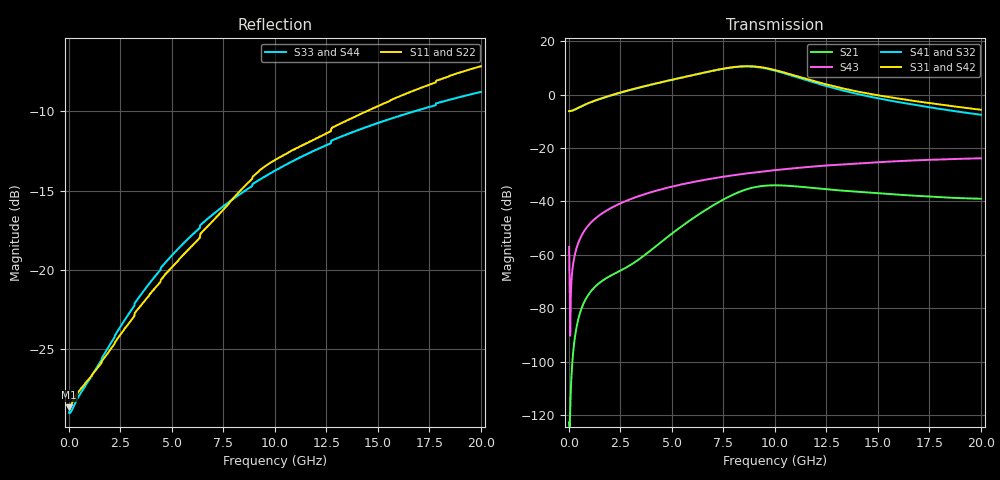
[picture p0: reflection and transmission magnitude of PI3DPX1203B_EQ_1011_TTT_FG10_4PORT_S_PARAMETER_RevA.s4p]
! NPort=4 DATA=2000 NOISE=0 GROUPDELAY=0 COMPLEX_DATAFORMAT=POLAR
! NumOfBlock=1 NumOfParam=0
! .MODEL Smodel S TSTONEFILE=PI3DPX1203B_EQ_1011_TTT_FG10_4PORT_S_PARAMETER_RevA.s4p TYPE=S
!  -- The above .MODEL line can be used for the S element in the netlist.
! The s parameter is extracted from the linear redriver, it is not bi-directional; only s(4,1)s(4,2) and s(3,1)s(3,2)
! should be the insertion loss
!Port definition:
!Port1 = input+
!Port2 = input-
!Port3 = output+
!Port4 = output-
# Hz S MA R  50
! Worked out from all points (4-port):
!   2000 points, 10 MHz to 20 GHz, reference 50 ohm
!   strongest paths, dB at 10 MHz, 5.01 GHz, 10.01 GHz, 15.01 GHz, 20 GHz:
!     S31: -6.2, 5.6, 9.2, -0.3, -5.7
!     S42: -6.2, 5.6, 9.2, -0.3, -5.7
!     S41: -6.2, 5.6, 9.0, -1.4, -7.6
!     S32: -6.2, 5.6, 9.0, -1.4, -7.6
!     S43: -57.1, -34.4, -28.3, -25.3, -23.8
!     S21: -122.7, -52.0, -34.0, -37.0, -39.0
!   lowest |S11| = -28.6 dB at 10 MHz (marker M1), VSWR 1.08, Z = 46.4 - j0.0306 ohm
!   |S11| at or under -10 dB: start of sweep to 14.45 GHz
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1e7  0.03701 -179.5  7.338e-07 10.7  0 0.0  0 0.0
     7.338e-07 10.7  0.03701 -179.5  0 0.0  0 0.0
     0.4917 -0.0  0.4917 180.0  0.03566 178.2  0.001403 -77.8
     0.4917 180.0  0.4917 -0.0  0.001403 -77.8  0.03566 178.2
3.08e9  0.07029 -126.9  0.0006803 139.5  1.482e-10 56.1  2.591e-09 107.3
        0.00068 139.5  0.07029 -126.9  2.591e-09 107.3  1.482e-10 56.1
        1.262 1.7  1.25 -177.1  0.07565 -126.7  0.01139 77.7
        1.25 -177.1  1.262 1.7  0.01139 77.7  0.07565 -126.7
5.82e9  0.1163 -111.0  0.004264 153.6  1.23e-08 -121.2  1.123e-07 69.2
        0.004263 153.6  0.1163 -111.0  1.123e-07 69.2  1.23e-08 -121.2
        2.235 -39.7  2.234 141.7  0.1263 -117.3  0.02225 66.0
        2.234 141.7  2.235 -39.7  0.02225 66.0  0.1263 -117.3
8.21e9  0.1749 -105.0  0.01475 111.0  3.09e-07 156.0  8.63e-07 20.0
        0.01474 111.0  0.1749 -105.0  8.622e-07 20.0  3.092e-07 156.0
        3.347 -98.7  3.316 82.5  0.1716 -115.9  0.03183 53.9
        3.317 82.5  3.346 -98.7  0.03183 53.9  0.1716 -115.9
9.75e9  0.2172 -107.2  0.01997 67.3  1.068e-06 94.8  1.812e-06 -17.6
        0.01996 67.3  0.2171 -107.2  1.81e-06 -17.6  1.069e-06 94.9
        3.045 -148.8  2.972 32.3  0.2012 -116.2  0.03759 45.7
        2.974 32.3  3.044 -148.8  0.03759 45.7  0.2012 -116.2
1.196e10  0.2584 -109.2  0.01776 26.3  2.838e-06 30.1  3.527e-06 -45.8
          0.01774 26.4  0.2584 -109.2  3.527e-06 -45.7  2.84e-06 30.1
          1.762 163.2  1.658 -15.5  0.2387 -117.4  0.04532 34.4
          1.659 -15.5  1.761 163.2  0.04532 34.4  0.2387 -117.4
2e10  0.4384 -117.6  0.01119 -17.6  2.238e-05 -109.1  3.137e-05 -133.8
      0.01124 -17.3  0.4385 -117.6  3.144e-05 -133.7  2.241e-05 -109.1
      0.5198 74.9  0.4192 -92.4  0.3637 -123.9  0.06431 -7.1
      0.419 -92.5  0.5205 75.0  0.06431 -7.1  0.3637 -123.9
